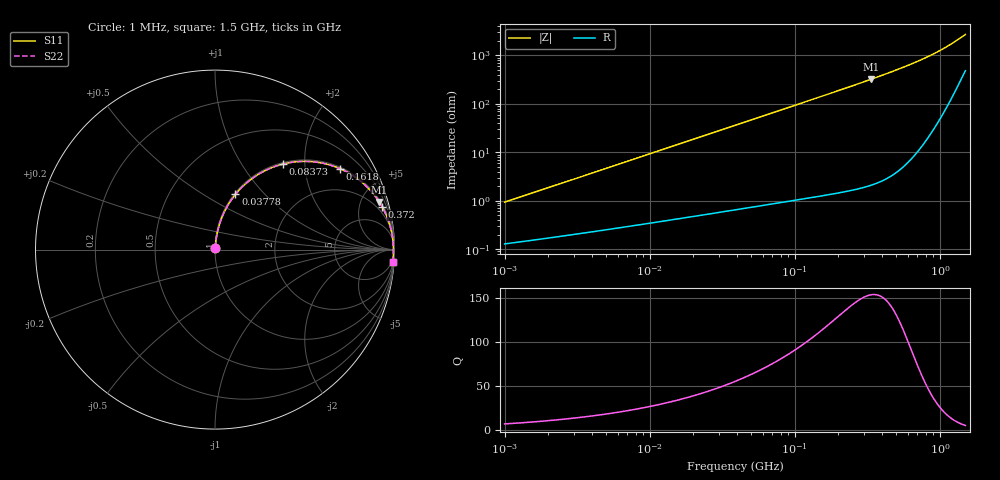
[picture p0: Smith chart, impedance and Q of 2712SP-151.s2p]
# MHz  S  MA  R  50
!Freq  MagS11  AngS11  MagS21  AngS21  MagS12  AngS12  MagS22  AngS22
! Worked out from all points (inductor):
!   801 points, 1 MHz to 1.5 GHz, reference 50 ohm
!   read as one part in series: L = 148 nH near 1.037 MHz
!   highest Q = 154 at 336.3 MHz (marker M1), where L = 153 nH
!   S11 on the Smith chart (normalised r, x): 1 MHz: 1.00, +0.02; 37.78 MHz: 1.01, +0.70; 83.73 MHz: 1.03, +1.56; 161.8 MHz: 1.05, +3.06; 372 MHz: 1.23, +7.76; 1.5 GHz: 3, -27
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1  0.009323 81.6  0.9987 -0.5  0.9987 -0.5  0.009323 81.6
3.407013  0.03149 84.3  0.9974 -1.8  0.9974 -1.8  0.03149 84.3
6.64352  0.06121 83.8  0.9953 -3.5  0.9953 -3.5  0.06121 83.8
11.50203  0.1054 81.9  0.9908 -6.1  0.9908 -6.1  0.1054 81.9
16.43309  0.1497 79.7  0.9845 -8.7  0.9845 -8.7  0.1497 79.7
22.84257  0.2058 76.7  0.9737 -11.9  0.9737 -11.9  0.2057 76.7
29.78243  0.2642 73.4  0.959 -15.4  0.959 -15.4  0.2642 73.4
37.77953  0.3281 69.7  0.9387 -19.3  0.9387 -19.3  0.3281 69.7
38.83072  0.3362 69.2  0.9358 -19.8  0.9358 -19.8  0.3362 69.2
57.02152  0.464 61.3  0.879 -27.8  0.879 -27.8  0.4639 61.3
83.73407  0.6095 51.5  0.7855 -37.8  0.7855 -37.8  0.6094 51.5
105.2509  0.6949 45.0  0.7117 -44.4  0.7117 -44.4  0.6949 45.0
131.092  0.7694 38.7  0.6315 -50.7  0.6315 -50.7  0.7693 38.7
161.7908  0.8301 32.9  0.5506 -56.6  0.5506 -56.6  0.83 32.9
231.1524  0.9059 23.9  0.4172 -65.7  0.4172 -65.7  0.9057 23.9
336.348  0.9532 16.1  0.2965 -73.5  0.2965 -73.5  0.953 16.1
371.9557  0.9616 14.3  0.2685 -75.3  0.2685 -75.3  0.9614 14.3
446.6321  0.9735 11.4  0.2223 -78.3  0.2223 -78.3  0.9733 11.4
649.8909  0.9879 6.1  0.1449 -83.2  0.1449 -83.2  0.9876 6.1
878.9161  0.993 2.4  0.09665 -86.1  0.09665 -86.1  0.9927 2.4
1114.92  0.9941 -0.4  0.06577 -87.1  0.06577 -87.1  0.994 -0.4
1500  0.9925 -4.1  0.03664 -83.8  0.03664 -83.8  0.9926 -4.1
